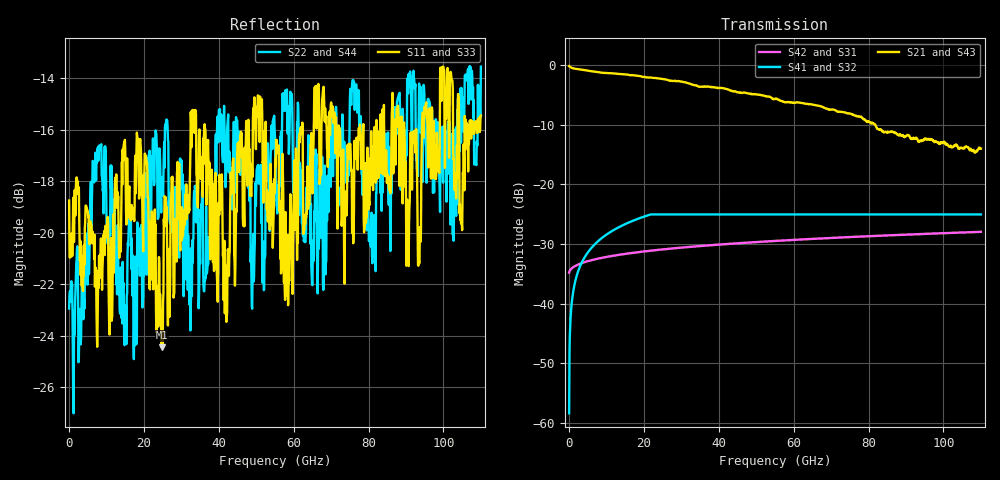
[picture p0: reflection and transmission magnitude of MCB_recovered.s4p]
! Created with skrf 1.10.0 (http://scikit-rf.org).
# GHz S RI R 50.0
!freq ReS11 ImS11 ReS12 ImS12 ReS13 ImS13
! ReS14 ImS14
! ReS21 ImS21 ReS22 ImS22 ReS23 ImS23
! ReS24 ImS24
! ReS31 ImS31 ReS32 ImS32 ReS33 ImS33
! ReS34 ImS34
! ReS41 ImS41 ReS42 ImS42 ReS43 ImS43
! ReS44 ImS44
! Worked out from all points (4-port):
!   1101 points, 10 MHz to 110 GHz, reference 50 ohm
!   strongest paths, dB at 10 MHz, 27.51 GHz, 55.01 GHz, 82.5 GHz, 110 GHz:
!     S21: -0.2, -2.6, -5.7, -10.7, -14.0
!     S43: -0.2, -2.7, -5.7, -10.6, -13.9
!     S41: -58.4, -25.0, -25.0, -25.0, -25.0
!     S32: -58.4, -25.0, -25.0, -25.0, -25.0
!     S42: -34.8, -30.8, -29.5, -28.6, -28.0
!     S31: -34.8, -30.8, -29.5, -28.6, -28.0
!   lowest |S11| = -24.4 dB at 24.71 GHz (marker M1), VSWR 1.13, Z = 48.1 + j5.58 ohm
!   |S11| at or under -10 dB: start of sweep to end of sweep
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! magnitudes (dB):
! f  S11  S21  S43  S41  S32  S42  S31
! 10 MHz  -18.7  -0.2  -0.2  -58.4  -58.4  -34.8  -34.8
! 1.01 GHz  -19.8  -0.5  -0.5  -38.4  -38.4  -33.9  -33.9
! 4.01 GHz  -20.5  -0.8  -0.9  -32.4  -32.4  -33.1  -33.1
! 24.71 GHz  -24.4  -2.3  -2.2  -25.0  -25.0  -30.9  -30.9
! 33.31 GHz  -15.3  -3.3  -3.2  -25.0  -25.0  -30.4  -30.4
! 41.81 GHz  -22.6  -4.0  -4.0  -25.0  -25.0  -30.0  -30.0
! 110 GHz  -15.4  -14.0  -13.9  -25.0  -25.0  -28.0  -28.0
